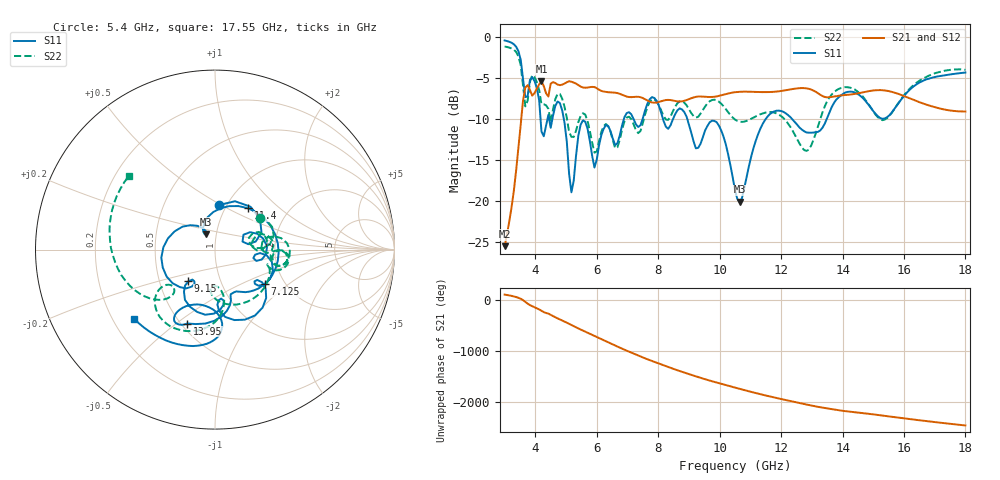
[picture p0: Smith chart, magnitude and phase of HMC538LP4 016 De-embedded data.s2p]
! Chelmsford, MA 01824
! http://www.hittite.com
! Tel: 978-250-3343
! Fax: 978-250-3373
! Device  :  HMC538LP4
! Description:  600 Analog Phase Shifter
! Frequency  :  6.0 GHz - 15.0 GHz
! Package  :  LP4  - 4x4 mm Quad Flatpack No-Lead (QFN) Plastic Package: 24 pin
! Ports  :  2 RF, 1 DC
!  Pin  3  = Rfin  = Port 1
!  Pin  16  = Rfout = Port 2
!  pin  21  = vCTL
! Voltages:  VCTL  = 0 to 5.0 Volts
! Currents :  Vb(V)  Vd(V)  Ib(mA)  Id(mA)
!  0.00  1.60  0.000000	0.490108
! Data:  The device was measured on evaluation board 111296-1.
!  Data was collected using a calibrated network analyzer.
!  The evaluation circuit board was modeled and simulated.This was use
!  to removed the evaluation board circuit from the measured data.
!  The reference plane is the center of the package pin.
! Misc:  Lot #
!Date Measured:  03 - 11 -2009
! Date:  03 - 17 -2009
! Note:
!  Hittite Microwave supplies this data as a sample of measured data at the
!  package pin for this package product.  Your particular data for this product
!  may vary.
!  Data was taken at 25 degrees C.
!  Hittite Microwave reserves the right to change this data at anytime.
# MHz S MA R 50
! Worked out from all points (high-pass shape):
!   201 points, 3 GHz to 18 GHz, reference 50 ohm
!   highest |S21| = -5.37 dB at 4.2 GHz (marker M1); lowest = -25.5 dB at 3 GHz (marker M2)
!   |S21| within 3 dB of the highest: 3.584 GHz to 16.83 GHz (13.25 GHz wide, 130 % of centre)
!   lowest |S11| = -20.1 dB at 10.65 GHz (marker M3), VSWR 1.22, Z = 44.5 + j7.59 ohm
!   |S11| at or under -10 dB: 4.928 GHz to 6.883 GHz (1.956 GHz wide, 33.1 % of centre); 8.946 GHz to 11.5 GHz (2.556 GHz wide, 25 % of centre); 12.36 GHz to 13.49 GHz (1.13 GHz wide, 8.75 % of centre)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
!   |S22| runs from -14.1 to -1.2 dB; largest |S21 - S12| = 0.0011
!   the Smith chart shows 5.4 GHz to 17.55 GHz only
!   S11 on the Smith chart (normalised r, x): 5.4 GHz: 0.92, +0.49; 7.125 GHz: 1.58, -0.69; 9.15 GHz: 0.70, -0.26; 11.4 GHz: 1.27, +0.64; 13.95 GHz: 0.54, -0.55; 17.55 GHz: 0.29, -0.34
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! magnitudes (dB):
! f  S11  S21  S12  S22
! 3 GHz  -0.4  -25.5  -25.5  -1.2
! 3.45 GHz  -1.7  -13.5  -13.5  -2.4
! 3.675 GHz  -7.3  -6.2  -6.2  -8.5
! 3.975 GHz  -5.4  -6.8  -6.8  -4.9
! 4.2 GHz  -11.5  -5.4  -5.4  -8.2
! 4.8 GHz  -8.1  -5.9  -5.9  -6.9
! 5.175 GHz  -19.0  -5.5  -5.5  -12.2
! 5.4 GHz  -12.0  -5.9  -5.9  -10.4
! 5.55 GHz  -10.2  -6.2  -6.2  -9.3
! 5.925 GHz  -15.9  -6.1  -6.1  -14.1
! 7.125 GHz  -9.4  -7.3  -7.3  -10.0
! 8.025 GHz  -8.4  -7.9  -7.9  -8.3
! 9.15 GHz  -12.7  -7.4  -7.4  -9.7
! 9.9 GHz  -10.4  -7.3  -7.3  -7.7
! 10.5 GHz  -18.7  -6.7  -6.7  -10.1
! 10.65 GHz  -20.1  -6.7  -6.7  -10.3
! 11.4 GHz  -10.6  -6.7  -6.7  -9.3
! 13.05 GHz  -11.7  -6.5  -6.5  -12.6
! 13.95 GHz  -7.1  -7.1  -7.1  -6.2
! 15.53 GHz  -9.6  -6.6  -6.6  -9.6
! 17.55 GHz  -4.5  -9.0  -9.0  -4.0
! 18 GHz  -4.3  -9.1  -9.1  -4.0
